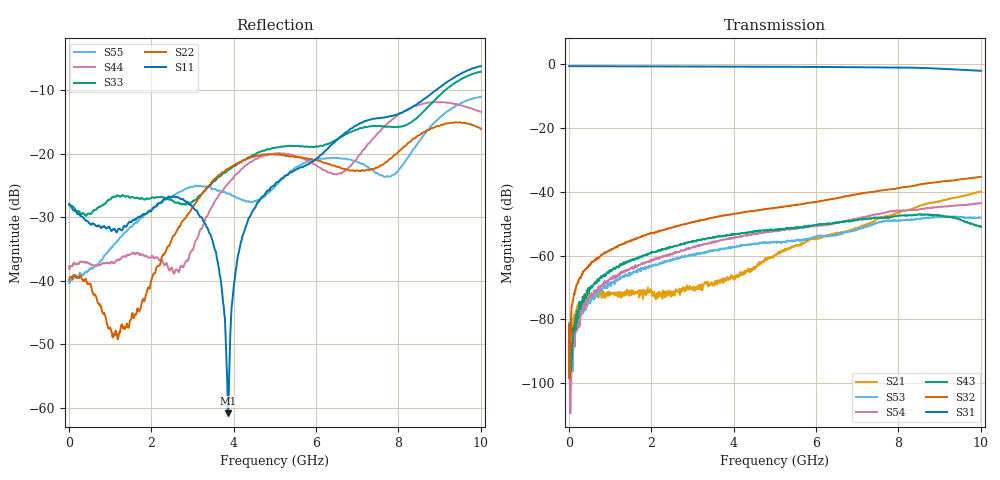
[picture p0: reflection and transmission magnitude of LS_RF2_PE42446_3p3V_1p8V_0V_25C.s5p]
! Created Wed Jan 31 17:16:06 2024
# ghz S ma R 50
! 5 Port Network Data from SP1.SP block
! freq  magS11  angS11  magS12  angS12  magS13  angS13  magS14  angS14
!  magS15  angS15
!  magS21  angS21  magS22  angS22  magS23  angS23
!  magS24  angS24  magS25  angS25
!  magS31  angS31  magS32  angS32
!  magS33  angS33  magS34  angS34  magS35  angS35
!  magS41  angS41
!  magS42  angS42  magS43  angS43  magS44  angS44  magS45  angS45
!  magS51  angS51  magS52  angS52  magS53  angS53  magS54  angS54
!  magS55  angS55
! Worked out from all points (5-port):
!   1000 points, 10 MHz to 10 GHz, reference 50 ohm
!   strongest paths, dB at 10 MHz, 2.51 GHz, 5.01 GHz, 7.51 GHz, 10 GHz:
!     S31: -0.6, -0.7, -0.7, -0.9, -2.0
!     S32: -81.6, -51.1, -45.0, -39.7, -35.3
!     S43: -81.9, -57.2, -51.9, -48.0, -50.9
!     S54: -89.5, -59.7, -52.3, -47.1, -43.5
!     S53: -81.1, -61.4, -55.7, -49.6, -48.0
!     S21: -84.5, -71.5, -59.7, -48.4, -39.9
!   lowest |S11| = -60.9 dB at 3.87 GHz (marker M1), VSWR 1.00, Z = 50.1 + j0.0661 ohm
!   |S11| at or under -10 dB: start of sweep to 8.911 GHz
